{attribute 'qualified_only'}
VAR_GLOBAL
//HW_IO
	CHAMBER_IN	AT	%I*	:CHAMBER_IN;
	CHAMBER_OUT	AT	%Q*	:CHAMBER_OUT;
	
	IGS_IN		AT	%I*	:IGS_IN;
	IGS_OUT		AT	%Q*	:IGS_OUT;
//MFC
	MFC_PV 		AT	%I*	:ARRAY [1..10] OF STR_FCSP700_INPUT;
	MFC_SV 		AT	%Q*	:ARRAY [1..10] OF STR_FCSP700_OUTPUT;

//EV
	EV1 		AT 	%Q*	:STR_EX260_SEC;

	EV2 		AT 	%Q*	:STR_EX260_SEC;

	EV3 		AT 	%Q*	:STR_EX260_SEC;

	EV4 		AT 	%Q*	:STR_EX260_SEC;
		
//APC VALVE
	APC_PV		AT 	%I*	:VAT_IN;
	APC_SV		AT 	%Q*	:VAT_OUT;

//TMP
	TURBO_SV	AT	%Q*	:TMP_OUT;

	TURBO_PV	AT 	%I*	:TMP_IN;
	
//CDG PG/VG
	VG103_PV	AT 	%I*	:STR_CDG200D;

	VG101_PV	AT 	%I*	:STR_CDG200D;

	VG102_PV	AT 	%I*	:STR_CDG200D;

	BA1_PV		AT 	%I*	:STR_BPG400;

	VG104_PV	AT 	%I*	:STR_CDG200D;

//CHILLER
	CHILLER1_PV	AT 	%I*	:CHILLER_IN;
	CHILLER1_SV	AT 	%Q*	:CHILLER_OUT;
	
	CHILLER2_PV	AT 	%I*	:CHILLER_IN;
	CHILLER2_SV	AT 	%Q*	:CHILLER_OUT;
END_VAR
